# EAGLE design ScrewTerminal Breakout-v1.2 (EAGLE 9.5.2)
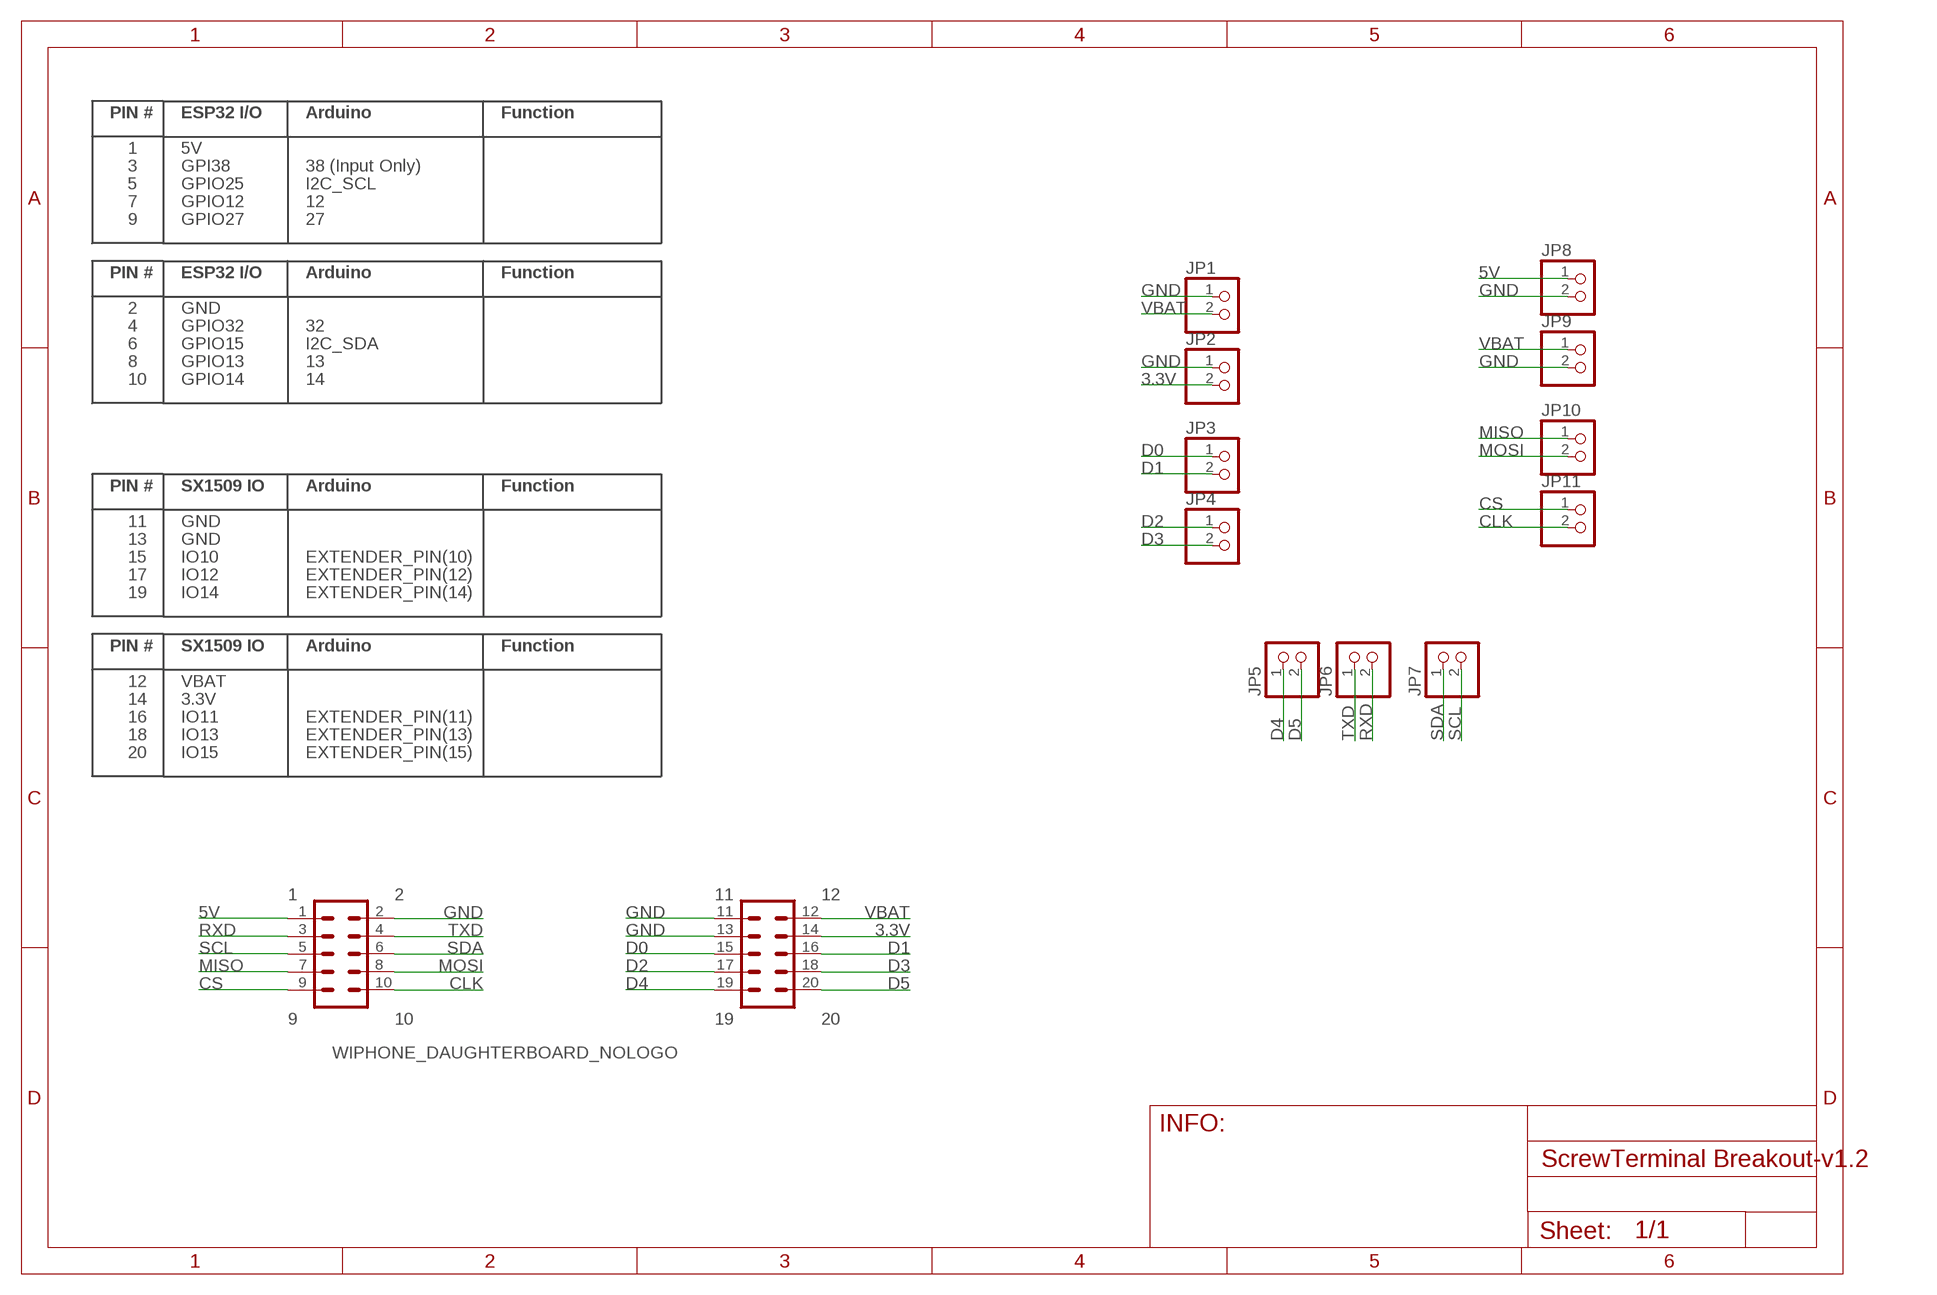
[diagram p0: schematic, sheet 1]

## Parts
JP1  SCREWTERMINAL-3.5MM-2  PINHD-1X2SCREWTERMINAL  [SCREWTERMINAL-3.5MM-2]
JP2  SCREWTERMINAL-3.5MM-2  PINHD-1X2SCREWTERMINAL  [SCREWTERMINAL-3.5MM-2]
JP3  SCREWTERMINAL-3.5MM-2  PINHD-1X2SCREWTERMINAL  [SCREWTERMINAL-3.5MM-2]
JP4  SCREWTERMINAL-3.5MM-2  PINHD-1X2SCREWTERMINAL  [SCREWTERMINAL-3.5MM-2]
JP5  SCREWTERMINAL-3.5MM-2  PINHD-1X2SCREWTERMINAL  [SCREWTERMINAL-3.5MM-2]
JP6  SCREWTERMINAL-3.5MM-2  PINHD-1X2SCREWTERMINAL  [SCREWTERMINAL-3.5MM-2]
JP7  SCREWTERMINAL-3.5MM-2  PINHD-1X2SCREWTERMINAL  [SCREWTERMINAL-3.5MM-2]
JP8  SCREWTERMINAL-3.5MM-2  PINHD-1X2SCREWTERMINAL  [SCREWTERMINAL-3.5MM-2]
JP9  SCREWTERMINAL-3.5MM-2  PINHD-1X2SCREWTERMINAL  [SCREWTERMINAL-3.5MM-2]
JP10  SCREWTERMINAL-3.5MM-2  PINHD-1X2SCREWTERMINAL  [SCREWTERMINAL-3.5MM-2]
JP11  SCREWTERMINAL-3.5MM-2  PINHD-1X2SCREWTERMINAL  [SCREWTERMINAL-3.5MM-2]
WIPHONE_DAUGHTERBOARD-FOOTPRINT1  WIPHONE_DAUGHTERBOARD_NOLOGO  [WIPHONE_DAUGHTERBOARD-NL]

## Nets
3.3V: JP2.2 WIPHONE_DAUGHTERBOARD-FOOTPRINT1.14
5V: JP8.1 WIPHONE_DAUGHTERBOARD-FOOTPRINT1.1
CLK: JP11.2 WIPHONE_DAUGHTERBOARD-FOOTPRINT1.10
CS: JP11.1 WIPHONE_DAUGHTERBOARD-FOOTPRINT1.9
D0: JP3.1 WIPHONE_DAUGHTERBOARD-FOOTPRINT1.15
D1: JP3.2 WIPHONE_DAUGHTERBOARD-FOOTPRINT1.16
D2: JP4.1 WIPHONE_DAUGHTERBOARD-FOOTPRINT1.17
D3: JP4.2 WIPHONE_DAUGHTERBOARD-FOOTPRINT1.18
D4: JP5.1 WIPHONE_DAUGHTERBOARD-FOOTPRINT1.19
D5: JP5.2 WIPHONE_DAUGHTERBOARD-FOOTPRINT1.20
GND: JP1.1 JP2.1 JP8.2 JP9.2 WIPHONE_DAUGHTERBOARD-FOOTPRINT1.2 WIPHONE_DAUGHTERBOARD-FOOTPRINT1.11 WIPHONE_DAUGHTERBOARD-FOOTPRINT1.13
MISO: JP10.1 WIPHONE_DAUGHTERBOARD-FOOTPRINT1.7
MOSI: JP10.2 WIPHONE_DAUGHTERBOARD-FOOTPRINT1.8
RXD: JP6.2 WIPHONE_DAUGHTERBOARD-FOOTPRINT1.3
SCL: JP7.2 WIPHONE_DAUGHTERBOARD-FOOTPRINT1.5
SDA: JP7.1 WIPHONE_DAUGHTERBOARD-FOOTPRINT1.6
TXD: JP6.1 WIPHONE_DAUGHTERBOARD-FOOTPRINT1.4
VBAT: JP1.2 JP9.1 WIPHONE_DAUGHTERBOARD-FOOTPRINT1.12

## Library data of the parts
JP1-JP11 = MZJ:PINHD-1X2: PIN HEADER
WIPHONE_DAUGHTERBOARD-FOOTPRINT1 = WiPhone:WIPHONE_DAUGHTERBOARD

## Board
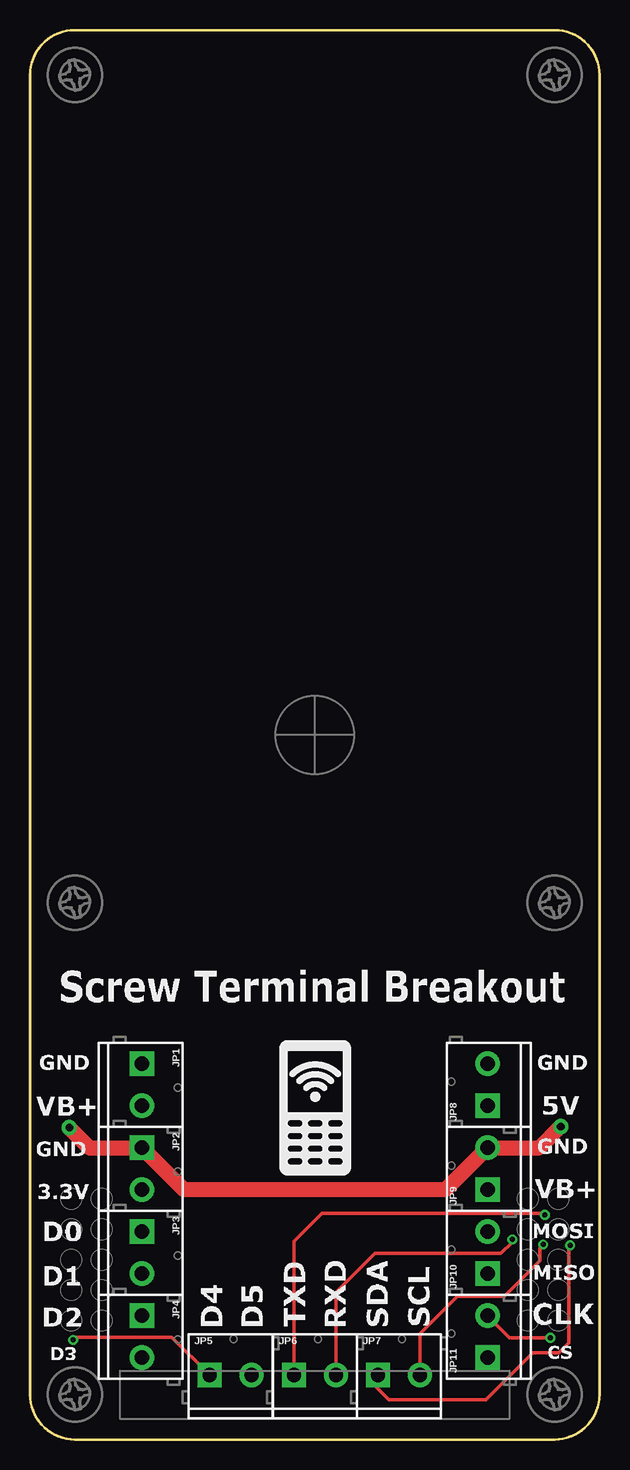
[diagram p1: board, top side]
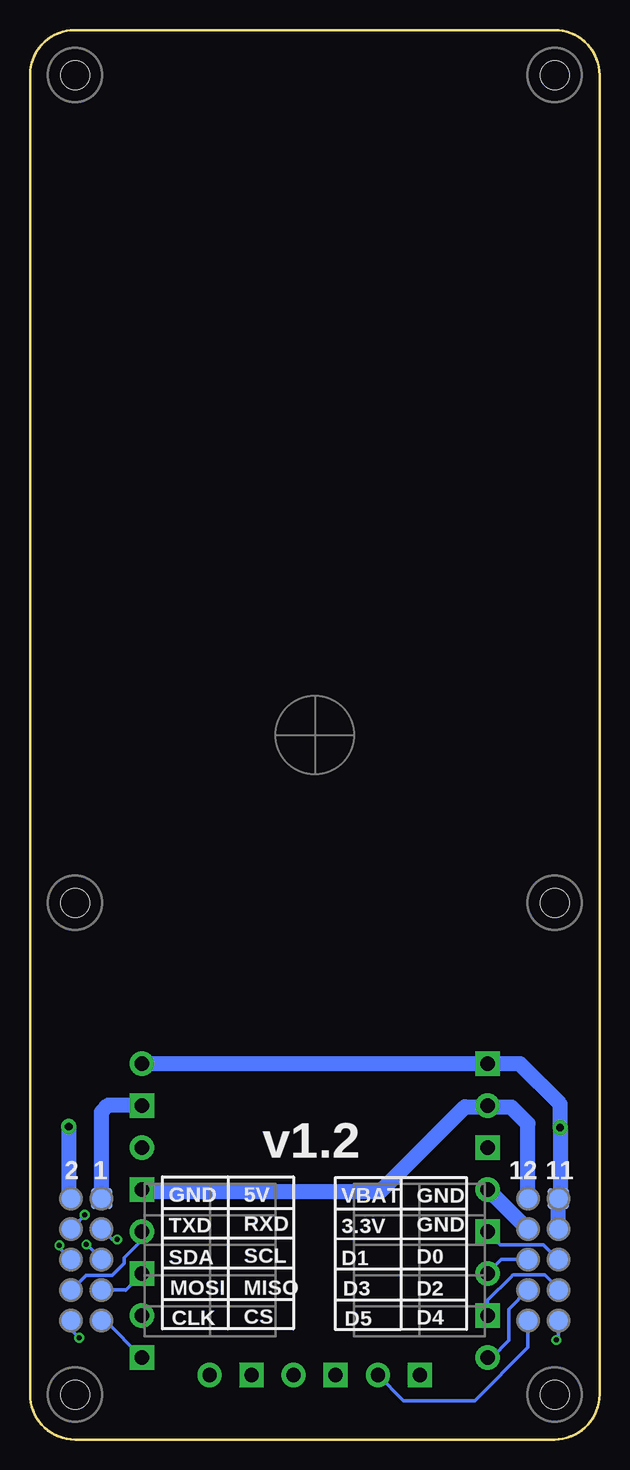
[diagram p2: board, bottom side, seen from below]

Size 47.5 x 117.5 mm. Coordinates in mm from the lower left corner, seen from the top.
Copper layers (1*16): Top 0.035mm / dielectric 1.5mm / Bottom 0.035mm
Design rules "2LDaughterBoards": minimum track width 6mil, minimum drill 6mil, track to track 8mil, track to pad 8mil, pad to pad 8mil, via to via 8mil, smd to smd 0mil, copper to edge 16mil, drill to drill 6mil, minimum pad ring 10mil, minimum via ring 8mil, stop-mask expansion 4mil, vias tented up to drill 25mil, thermal gap 10mil

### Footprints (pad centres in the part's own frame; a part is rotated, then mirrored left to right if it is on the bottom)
SCREWTERMINAL-3.5MM-2 = drill 1.2 pad 2.032 square: 1 0,0 | drill 1.2 pad 2.032: 2 3.5,0
WIPHONE_DAUGHTERBOARD-NL = smd 1.75 x 1.75 bottom: 1 17.78,-38.66; 2 20.32,-38.66; 3 17.78,-41.2; 4 20.32,-41.2; 5 17.78,-43.74; 6 20.32,-43.74; 7 17.78,-46.28; 8 20.32,-46.28; 9 17.78,-48.82; 10 20.32,-48.82; 11 -20.32,-38.66; 12 -17.78,-38.66; 13 -20.32,-41.2; 14 -17.78,-41.2; 15 -20.32,-43.74; 16 -17.78,-43.74; 17 -20.32,-46.28; 18 -17.78,-46.28; 19 -20.32,-48.82; 20 -17.78,-48.82 | hole 2.4: 20,-54.991; -20,-54.991; 20,-13.991; 20,55.009; -20,55.009; -20,-13.991

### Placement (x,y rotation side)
JP1  9.34,31.33 270 top
JP2  9.34,24.33 270 top
JP3  9.34,17.33 270 top
JP4  9.34,10.33 270 top
JP5  14.98,5.38 0 top
JP6  22.02,5.38 0 top
JP7  29.02,5.38 0 top
JP8  38.15,27.83 90 top
JP9  38.15,20.83 90 top
JP10  38.15,13.83 90 top
JP11  38.15,6.83 90 top
WIPHONE_DAUGHTERBOARD-FOOTPRINT1  23.75,58.74 0 top

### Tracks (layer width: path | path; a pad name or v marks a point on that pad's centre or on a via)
3.3V
  Bottom 1.27: WIPHONE_DAUGHTERBOARD-FOOTPRINT1.14 9.26,20.83 JP2.2
5V
  Bottom 1.27: WIPHONE_DAUGHTERBOARD-FOOTPRINT1.1 41.53,27.31 40.96,27.88 38.21,27.88 JP8.1
CLK  (via drill 0.41)
  Top 0.305: v43.39,8.48 40,8.48 JP11.2
  Bottom 0.305: WIPHONE_DAUGHTERBOARD-FOOTPRINT1.10 44.07,9.16 v43.39,8.48
CS
  Bottom 0.305: JP11.1 41.24,9.92 WIPHONE_DAUGHTERBOARD-FOOTPRINT1.9
D0
  Bottom 0.305: JP3.1 8.25,16.24 4.67,16.24 WIPHONE_DAUGHTERBOARD-FOOTPRINT1.15
D1
  Bottom 0.305: WIPHONE_DAUGHTERBOARD-FOOTPRINT1.16 8.17,15 JP3.2
D2
  Bottom 0.305: JP4.1 9.34,11.59 7.37,13.56 7.25,13.68 7.19,13.74 4.55,13.74 3.43,12.62 WIPHONE_DAUGHTERBOARD-FOOTPRINT1.17
D3
  Bottom 0.305: JP4.2 8.99,6.83 7.56,8.26 7.56,10.87 WIPHONE_DAUGHTERBOARD-FOOTPRINT1.18
D4  (via drill 0.41)
  Top 0.305: JP5.1 11.82,8.54 3.84,8.54 v3.6,8.3
  Bottom 0.305: WIPHONE_DAUGHTERBOARD-FOOTPRINT1.19 3.43,8.47 v3.6,8.3
D5
  Bottom 0.305: JP5.2 16.34,3.24 10.41,3.24 5.96,7.69 WIPHONE_DAUGHTERBOARD-FOOTPRINT1.20
GND  (via drill 0.64 pad 1.27)
  Top 1.27: v3.28,25.99 4.99,24.28 9.39,24.28 JP2.1 12.84,20.83 34.65,20.83 JP9.2 42.51,24.33 v44.27,26.09
  Bottom 1.27: WIPHONE_DAUGHTERBOARD-FOOTPRINT1.13 WIPHONE_DAUGHTERBOARD-FOOTPRINT1.11 3.28,20.23 v3.28,25.99 3.28,27.97 6.64,31.33 JP1.1 JP8.2 | WIPHONE_DAUGHTERBOARD-FOOTPRINT1.2 44.27,20.28 v44.27,26.09
MISO
  Bottom 0.305: JP10.1 39.53,12.45 39.54,12.46 WIPHONE_DAUGHTERBOARD-FOOTPRINT1.7
MOSI
  Bottom 0.305: JP10.2 38.15,16.64 39.65,15.14 39.65,14.68 40.64,13.69 42.83,13.69 WIPHONE_DAUGHTERBOARD-FOOTPRINT1.8
RXD  (via drill 0.41)
  Top 0.305: v40.22,16.67 40.22,16.45 39.28,15.51 28.78,15.51 25.52,12.25 JP6.2
  Bottom 0.305: WIPHONE_DAUGHTERBOARD-FOOTPRINT1.3 40.66,16.67 v40.22,16.67
SCL  (via drill 0.41)
  Top 0.305: JP7.2 32.52,8.81 35.65,11.94 39.55,11.94 42.5,14.89 42.5,15.96 v42.8,16.26
  Bottom 0.305: WIPHONE_DAUGHTERBOARD-FOOTPRINT1.5 42.78,16.26 v42.8,16.26
SDA  (via drill 0.41)
  Top 0.305: JP7.1 28.87,5.23 28.87,4.4 29.94,3.33 38.04,3.33 41.94,7.23 44.12,7.23 44.95,8.06 44.95,16.1 v45.05,16.2
  Bottom 0.305: WIPHONE_DAUGHTERBOARD-FOOTPRINT1.6 45.05,15.98 v45.05,16.2
TXD  (via drill 0.41)
  Top 0.305: JP6.1 22.02,16.53 24.35,18.86 42.81,18.86 v42.94,18.73
  Bottom 0.305: WIPHONE_DAUGHTERBOARD-FOOTPRINT1.4 42.94,18.67 v42.94,18.73
VBAT
  Bottom 1.27: 9.25,27.74 JP1.2 | JP9.1 arc-90 38.02,20.7 18.27,20.7 11.23,27.74 9.25,27.74 | 9.25,27.74 9.21,27.69 7.35,27.69 5.97,26.31 WIPHONE_DAUGHTERBOARD-FOOTPRINT1.12

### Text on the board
bPlace: v1.2 | GND | VBAT | 5V | GND | GND | RXD | TXD | 3.3V | D0 | D1 | SCL | SDA | D2 | D3 | MISO | MOSI | D4 | D5 | CS | CLK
